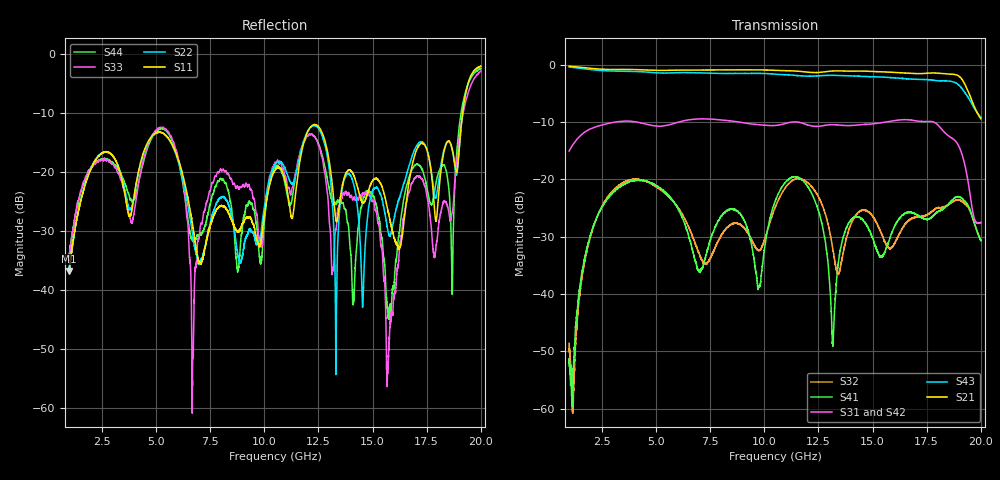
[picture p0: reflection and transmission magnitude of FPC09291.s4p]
!The following data was pulled from an Agilent PNA
!This sNp file was generated from the data in the RF Test software
!NOTE:  Smoothing/Math/Corrections applied on any given trace ARE included in the data saved here
# MHz S dB R 50
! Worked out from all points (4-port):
!   6401 points, 1 GHz to 20 GHz, reference 50 ohm
!   strongest paths, dB at 1 GHz, 5.75 GHz, 10.5 GHz, 15.25 GHz, 20 GHz:
!     S21: -0.3, -1.0, -1.0, -1.2, -9.4
!     S43: -0.4, -1.4, -1.6, -2.1, -9.2
!     S31: -15.1, -10.3, -10.6, -10.2, -27.5
!     S42: -15.1, -10.4, -10.7, -10.2, -27.2
!     S41: -51.9, -23.6, -23.9, -32.7, -30.7
!     S32: -48.6, -23.6, -25.0, -28.2, -30.6
!   lowest |S11| = -36.7 dB at 1 GHz (marker M1), VSWR 1.03, Z = 51.4 - j0.449 ohm
!   |S11| at or under -10 dB: start of sweep to 19.15 GHz
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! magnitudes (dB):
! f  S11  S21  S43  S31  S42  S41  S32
! 1 GHz  -36.7  -0.3  -0.4  -15.1  -15.1  -51.9  -48.6
! 3.342 GHz  -19.9  -0.8  -1.1  -9.9  -10.0  -21.3  -20.9
! 5.67 GHz  -14.7  -1.0  -1.4  -10.4  -10.5  -23.2  -23.3
! 6.712 GHz  -29.3  -0.9  -1.4  -9.5  -9.6  -32.6  -30.2
! 12.16 GHz  -12.3  -1.3  -2.0  -10.7  -10.7  -22.2  -21.1
! 15.72 GHz  -26.6  -1.3  -2.2  -9.9  -9.9  -31.2  -31.9
! 20 GHz  -2.0  -9.4  -9.2  -27.5  -27.2  -30.7  -30.6
